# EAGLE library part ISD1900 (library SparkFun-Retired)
Voice recorder IC Retired IC -- Limited supply available
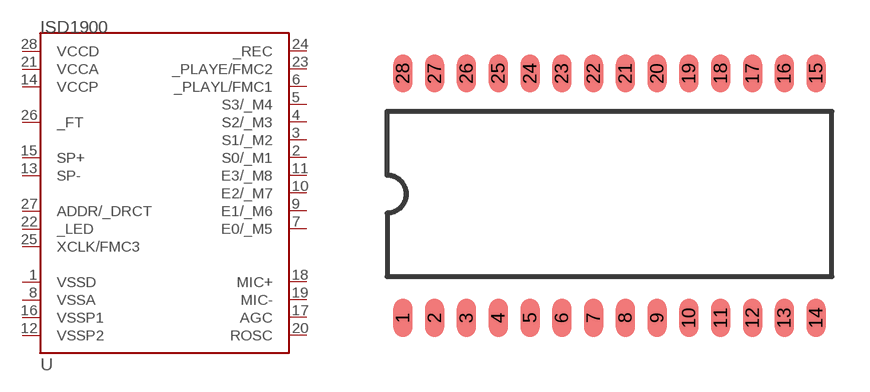
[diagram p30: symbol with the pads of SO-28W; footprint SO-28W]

Designator prefix U

## ISD1900ISD1932  [SO-28W]
1  VSSD
2  S0/_M1
3  S1/_M2
4  S2/_M3
5  S3/_M4
6  _PLAYL/FMC1
7  E0/_M5
8  VSSA
9  E1/_M6
10  E2/_M7
11  E3/_M8
12  VSSP2
13  SP-
14  VCCP
15  SP+
16  VSSP1
17  AGC
18  MIC+
19  MIC-
20  ROSC
21  VCCA
22  _LED
23  _PLAYE/FMC2
24  _REC
25  XCLK/FMC3
26  _FT
27  ADDR/_DRCT
28  VCCD

## Footprint SO-28W (pad centres in mm)
Small Outline Wide Plastic Gull Wing 300-mil body, package type SO
smd 0.762 x 1.524: 1 -8.255,-4.953; 2 -6.985,-4.953; 3 -5.715,-4.953; 4 -4.445,-4.953; 5 -3.175,-4.953; 6 -1.905,-4.953; 7 -0.635,-4.953; 8 0.635,-4.953; 9 1.905,-4.953; 10 3.175,-4.953; 11 4.445,-4.953; 12 5.715,-4.953; 13 6.985,-4.953; 14 8.255,-4.953; 15 8.255,4.826; 16 6.985,4.826; 17 5.715,4.826; 18 4.445,4.826; 19 3.175,4.826; 20 1.905,4.826; 21 0.635,4.826; 22 -0.635,4.826; 23 -1.905,4.826; 24 -3.175,4.826; 25 -4.445,4.826; 26 -5.715,4.826; 27 -6.985,4.826; 28 -8.255,4.826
